VAR_GLOBAL
	engine		AT %QX0.0:	BOOL;
	deviceUp	AT %QX0.1:	BOOL;
	deviceDown	AT %QX0.2:	BOOL;
	timerUp:					TON;
	timerDown:				TON;
	steps:					BYTE;
	count:					UINT := 0;
	devSpeed:				TIME := t#10ms;
	devTimer:				TON;
	switch: BOOL;
END_VAR
